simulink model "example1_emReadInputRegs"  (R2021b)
settings: Solver=FixedStepAuto  StartTime=0  StopTime=inf  FixedStep=0.5  RelTol=1e-3  EnableMultiTasking=on
undefined symbols (not defined in the file or in its folder): based, classic, dsPic33, MCC, Microchip, PIC24
libraries: emMBSlaveLib x4, simulink x1, embeddedCreatorLib x1

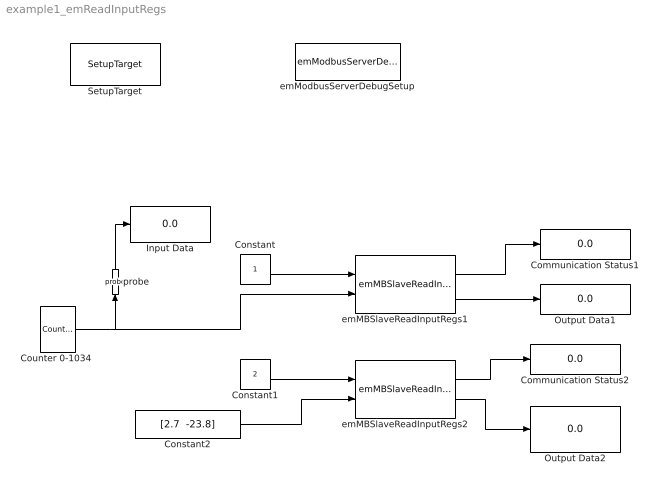
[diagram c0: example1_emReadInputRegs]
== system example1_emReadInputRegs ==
  Communication Status1 : Display
  Communication Status2 : Display
  Constant : Constant  OutDataTypeStr=uint16
  Constant1 : Constant  Value=2  OutDataTypeStr=uint16
  Constant2 : Constant  Value="[2.7  -23.8]"  OutDataTypeStr=single
  "Counter 0-1034 " : simulink/Sources/Counter Limited  uplimit=1034  tsamp=-1
  Input Data : Display
  Output Data1 : Display
  Output Data2 : Display
  SetupTarget : embeddedCreatorLib/SetupTarget  Tag=SetupTarget  Priority=0  c_platform=Microchip PIC24/dsPic33 based on MCC classic  c_debug=on
  emMBSlaveReadInputRegs1 : emMBSlaveLib/emMBSlaveReadInputRegs  c_ServerID=1  c_OutputDataType=uint16  c_wordOrder=big-endian  c_factor=1x  c_minAdr=1  c_RegQTY=10  c_InPortDataType=uint16  c_sampleTime=-1
  emMBSlaveReadInputRegs2 : emMBSlaveLib/emMBSlaveReadInputRegs  c_ServerID=1  c_OutputDataType=int32  c_wordOrder=big-endian  c_factor=10x  c_minAdr=1  c_RegQTY=10  c_InPortDataType=single  c_sampleTime=-1
  emModbusServerDebugSetup : emMBSlaveLib/emModbusServerDebugSetup  Tag=emModbusSlaveSetup  c_objID=0  c_uartNo=2  c_baudrate=19200  c_serverID=1  c_baudrate4PC=19200  c_forceLongerSpace=on  c_holdingRegsQTY=0  c_minHoldingAddr=789  c_inputRegsQTY=10  c_minInputRegAddr=1  c_coilRegsQTY=0  c_minCoilAddr=30  c_discreteRegsQTY=0  c_minDiscreteAddr=40  c_enableDebug=on  c_breakpointMaxQTY=100  c_probeMaxWordQTY=200  c_emWaitQTY=0  g_COMPortNo=COM5  c_Name_method=By physical port name and bit number  c_PortName=B  c_BitNo=11  c_TxEnable485="\"LATBbits.LATB11\""  c_TxEnable485Polarity=on
  probe : emMBSlaveLib/probe  Tag=emProbe  c_ObjID=0  c_serverID=1  c_UartNo=2  c_StartAddr=2  c_ConstantDataSource=off
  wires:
  Constant/1 -> emMBSlaveReadInputRegs1/1
  emMBSlaveReadInputRegs1/1 -> Communication Status1/1
  "Counter 0-1034 "/1 -> probe/1, emMBSlaveReadInputRegs1/2
  emMBSlaveReadInputRegs1/2 -> Output Data1/1
  probe/1 -> Input Data/1
  Constant1/1 -> emMBSlaveReadInputRegs2/1
  emMBSlaveReadInputRegs2/1 -> Communication Status2/1
  emMBSlaveReadInputRegs2/2 -> Output Data2/1
  Constant2/1 -> emMBSlaveReadInputRegs2/2
